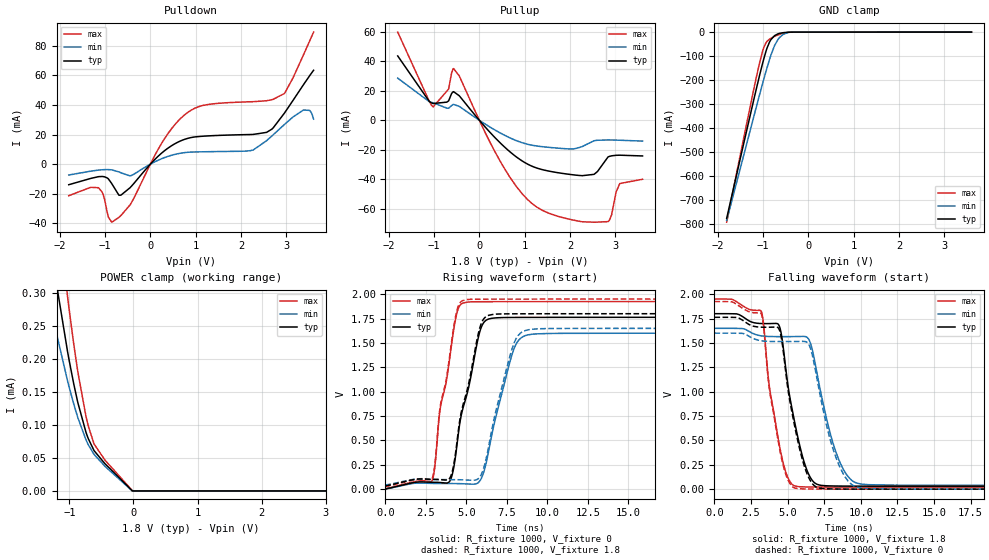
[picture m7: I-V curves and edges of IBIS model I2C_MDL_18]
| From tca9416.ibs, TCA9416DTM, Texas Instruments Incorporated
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[Model]   I2C_MDL_18
Model_type   I/O
Polarity   Non-Inverting
Enable   Active-High
Vinl = 0.54
Vinh = 1.26
Vmeas = 0.9
Vref = 0
Cref = 2pF
Rref = 100000
|   typ   min   max
C_comp   7.2608pF   6.6746pF   7.8469pF
[Voltage Range]   1.8   1.62   1.98
[Temperature Range]   27   125   -40
[Pullup Reference]   1.8   1.62   1.98
[Pulldown Reference]   0   0   0
[Power Clamp Reference]   1.8   1.62   1.98
[GND Clamp Reference]   0   0   0
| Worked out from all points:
|   slope of the pulldown table from 0 to 0.27 V, typ, clamps not added: 33.7 ohm
|   slope of the pullup table from 0 to 0.27 V, typ, clamps not added: 29 ohm
|   GND clamp passes 1 mA (typ) near -0.46 V on its own axis
|   rising waveform, R_fixture 1000, V_fixture 0: 20-80 % time 1.22ns typ, 1.36ns min, 990ps max; typ from 0.001 V to 1.76 V
|   falling waveform, R_fixture 1000, V_fixture 1.8: 20-80 % time 1.22ns typ, 1.51ns min, 1.06ns max; typ from 1.8 V to 0.031 V
|   rising waveform, R_fixture 1000, V_fixture 1.8: 20-80 % time 1.21ns typ, 1.34ns min, 987ps max; typ from 0.031 V to 1.8 V
|   falling waveform, R_fixture 1000, V_fixture 0: 20-80 % time 1.22ns typ, 1.49ns min, 1.05ns max; typ from 1.76 V to 0.001 V
[Pulldown]
|I2C_MDL_18
|   Voltage   I(typ)   I(min)   I(max)
-1.8V     -13.91mA   -7.35mA    -21.33mA
-1.147V   -8.486mA   -4.04mA    -15.94mA
-849.6mV  -13.3mA    -3.861mA   -39.25mA
-649.8mV  -20.97mA   -5.85mA    -34.77mA
257.4mV   7.701mA    3.78mA     14.54mA
689.4mV   16.01mA    7.509mA    31.53mA
1.143V    18.85mA    8.337mA    39.56mA
2.255V    20.09mA    9.473mA    42.22mA
2.682V    23.71mA    19.09mA    43.61mA
2.957V    34.53mA    26.84mA    47.76mA
3.379V    53.81mA    36.61mA    74.02mA
3.6V      63.48mA    30.42mA    89.29mA
[GND Clamp]
|I2C_MDL_18
|   Voltage   I(typ)   I(min)   I(max)
-1.8V     -776.5mA   -785.2mA   -792.6mA
-1.206V   -285.1mA   -355.3mA   -241.4mA
-1.076V   -181.9mA   -262.5mA   -129.8mA
-1.012V   -133.1mA   -217.1mA   -81.94mA
-984.6mV  -113.8mA   -198.6mA   -65.83mA
-930.6mV  -78.48mA   -162.2mA   -43.93mA
-855mV    -41.46mA   -114.3mA   -29.37mA
-747mV    -15.41mA   -57.54mA   -18.33mA
-666mV    -6.995mA   -30.24mA   -11.76mA
-558mV    -2.592mA   -9.815mA   -5.038mA
-444.6mV  -663.7uA   -1.401mA   -1.23mA
3.6V      0A         0A         0A
[Pullup]
|I2C_MDL_18
|   Voltage   I(typ)   I(min)   I(max)
-1.8V     43.54mA    28.52mA    59.7mA
-1.022V   11.37mA    11.85mA    9.156mA
-676.8mV  13.17mA    8.132mA    21.22mA
-568.8mV  19.37mA    10.73mA    35mA
538.2mV   -17.61mA   -9.865mA   -31.85mA
1.294V    -32.62mA   -17.54mA   -59.3mA
2.077V    -36.97mA   -19.39mA   -67.62mA
2.531V    -36.62mA   -13.87mA   -69.02mA
2.839V    -24.85mA   -13.33mA   -68.64mA
2.914V    -24.1mA    -13.37mA   -64.32mA
3.098V    -23.66mA   -13.53mA   -42.84mA
3.6V      -24.17mA   -14.11mA   -39.96mA
[POWER Clamp]
|I2C_MDL_18
|   Voltage   I(typ)   I(min)   I(max)
-1.8V     777.7uA    407.5uA    1.108mA
-1.363V   426.7uA    316.2uA    606.4uA
-1.184V   304.2uA    232.1uA    430.1uA
-1.028V   211.3uA    166.9uA    294.7uA
-936mV    164.6uA    133.4uA    226uA
-865.8mV  133.3uA    110.7uA    179.6uA
-741.6mV  89.26uA    77.79uA    113.5uA
-703.8mV  79.1uA     69.95uA    98.06uA
-617.4mV  61.69uA    55.82uA    72.14uA
-444.6mV  41.29uA    37.39uA    46.71uA
-23.4mV   636.3nA    377.6nA    970.2nA
3.6V      0A         0A         0A
[Ramp]
|I2C_MDL_18
| variable   typ   min   max
dV/dt_r   1.06/1.22E-09   0.96/1.36E-09   1.15/9.94E-10
dV/dt_f   1.06/1.22E-09   0.97/1.51E-09   1.16/1.06E-09
R_load = 1000
[Rising Waveform]
|I2C_MDL_18
R_fixture =   1000
C_fixture =   0
L_fixture =   0
V_fixture =   0
V_fixture_min = 0
V_fixture_max = 0
|   Time   V(typ)   V(min)   V(max)
0s        754.2uV    859.6uV    613uV
2.909ns   71.23mV    59.4mV     99.19mV
3.349ns   69.12mV    58.51mV    787.7mV
3.965ns   81.21mV    58.22mV    1.337V
4.361ns   378.4mV    57.87mV    1.769V
5.241ns   1.124V     52.6mV     1.921V
6.165ns   1.726V     230.6mV    1.923V
7.969ns   1.762V     1.451V     1.924V
9.377ns   1.762V     1.593V     1.924V
219.7ns   1.763V     1.6V       1.924V
[Falling Waveform]
|I2C_MDL_18
R_fixture =   1000
C_fixture =   0
L_fixture =   0
V_fixture =   1.8
V_fixture_min = 1.65
V_fixture_max = 1.95
|   Time   V(typ)   V(min)   V(max)
0s        1.8V       1.65V      1.95V
3.217ns   1.699V     1.572V     1.819V
3.745ns   1.698V     1.566V     1.062V
4.449ns   1.667V     1.565V     443mV
5.065ns   1.022V     1.565V     104.4mV
5.857ns   429.1mV    1.567V     25.47mV
6.605ns   107.7mV    1.476V     22.72mV
8.629ns   32.37mV    258mV      21.66mV
10.52ns   31.43mV    46.51mV    21.53mV
219.7ns   31.1mV     41.04mV    21.41mV
[Rising Waveform]
|I2C_MDL_18
R_fixture =   1000
C_fixture =   0
L_fixture =   0
V_fixture =   1.8
V_fixture_min = 1.65
V_fixture_max = 1.95
|   Time   V(typ)   V(min)   V(max)
0s        31.1mV     41.04mV    21.41mV
2.909ns   101.4mV    99.45mV    120.1mV
3.349ns   99.33mV    98.51mV    808.8mV
3.965ns   111.6mV    98.14mV    1.365V
4.361ns   410.7mV    97.75mV    1.796V
5.241ns   1.165V     92.6mV     1.947V
6.165ns   1.764V     274.2mV    1.949V
7.969ns   1.799V     1.508V     1.95V
9.553ns   1.799V     1.646V     1.95V
219.7ns   1.8V       1.65V      1.95V
[Falling Waveform]
|I2C_MDL_18
R_fixture =   1000
C_fixture =   0
L_fixture =   0
V_fixture =   0
V_fixture_min = 0
V_fixture_max = 0
|   Time   V(typ)   V(min)   V(max)
0s        1.763V     1.6V       1.924V
3.217ns   1.662V     1.522V     1.794V
3.745ns   1.661V     1.516V     1.037V
4.449ns   1.629V     1.514V     417.5mV
5.065ns   982.9mV    1.514V     82.5mV
5.857ns   391.2mV    1.516V     4.598mV
6.561ns   86.12mV    1.444V     1.97mV
8.585ns   2.054mV    221.9mV    857.6uV
10.48ns   1.087mV    6.3mV      729.1uV
219.7ns   754.2uV    859.6uV    613.1uV
